|Texas Instruments Incorporated
| IBIS Model of : TMUX7211
| 48V 4x1:1 Analog Switch Array
| This file contains package information for the following:
|  TSSOP 16-pin (PW) package as [Component] TMUX7211_PW
|  QFN 16-pin (RUM) package as [Component] TMUX7211_RUM
| This device can be powered at the following Vccs:
| Single Rail Supply Configurations:
|  5.0 volt VDD, 0V VSS
|  12.0 volt VDD, 0V VSS
|  36.0 volt VDD, 0V VSS
|  44.0 volt VDD, 0V VSS
| Dual Rail Supply Configurations:
|  5.0 volt VDD, -5V VSS
|  15.0 volt VDD, -15V VSS
|  20.0 volt VDD, -20V VSS
| Digital Voltage Range : 4.5-48.4
[IBIS Ver] 4.1
[File name] tmux7211.ibs
[File Rev] 1.0
[Date] 12/09/2020
[Source]
| Texas Instruments Incorporated.
| 12500 TI Blvd
| Dallas, TX -75243
[Notes] Revision History:
| Rev 1.0: 12/09/2020
| - Initial version of the model
| - Model generated from simulations in TISPICE/SPECTRE
| - C_comp although listed in numerical order of value are
| obtained from varying PVT conditions. For PVT conditions for
| each specific value refer the buffer description under
| respective [Model]. IBIS model user is responsible for using
| appropriate C_comp to simulate for Signal Integrity.
| - Warnings regarding combined Non-monotonicity of various models have been
| reviewed and considered minor and can be ignored.
|**** Modify the following if you use [Model Selector]***********
| - Model names with a trailing voltage extension contain the model for
| operation at that voltage range.
[Disclaimer]
| This model is designed as an aid for customers of Texas Instruments.
| TI and its licensors and suppliers make no warranties, either expressed
| or implied, with respect to this model, including the warranties of
| merchantability or fitness for a particular purpose. The model is
| provided solely on an "as is" basis. The entire risk as to its quality
| and performance is with the customer.
| This model is subject to change without notice. Texas Instruments
| Incorporated is not responsible for updating this model.
[Copyright]
(C) Copyright 2020 Texas Instruments Incorporated. All rights reserved.
| Component TMUX7211_DGK 8-pin SOT (per package)
[Component] TMUX7211_PW
[Manufacturer]  Texas Instruments Incorporated
[Package] |TSSOP (PW) 16-pin
| variable typ min max
R_pkg 0.05 0.04 0.06
L_pkg 1.0nH 0.8nH 1.2nH
C_pkg 0.2pF 0.16pF 0.24pF
| pin number (pin name) mapping to model name
[Pin] signal_name   model_name   R_pin L_pin C_pin
1   IN1 		INPUT_PD   NA   NA   NA
2   D1   TMUX7211_DX   NA   NA   NA
3   S1   TMUX7211_SX   NA   NA   NA
4   VSS   POWER   NA   NA   NA
5   GND 		GND   NA   NA   NA
6   S4   TMUX7211_SX   NA   NA   NA
7   D4   TMUX7211_DX   NA   NA   NA
8   IN4 		INPUT_PD   NA   NA   NA
9   IN3 		INPUT_PD   NA   NA   NA
10   D3   TMUX7211_DX   NA   NA   NA
11   S3   TMUX7211_SX   NA   NA   NA
12   NC   NC   NA   NA   NA
13   VDD 		POWER   NA   NA   NA
14   S2   TMUX7211_SX   NA   NA   NA
15   D2   TMUX7211_DX   NA   NA   NA
16   IN2 		INPUT_PD   NA   NA   NA
[Series Switch Groups]
| Function Group States
On  1 /   | S1->D1 IN HIGH
Off  /   | EN LOW
[Series Pin Mapping]   pin_2   model_name   function_table_group
| PW Package
|2   3   TMUX7211_SX_SINGLE_5V_S   1
|3   2   TMUX7211_DX_SINGLE_5V_S   1
|15   14   TMUX7211_SX_SINGLE_5V_S   1
|14   15   TMUX7211_DX_SINGLE_5V_S   1
|7   6   TMUX7211_SX_SINGLE_5V_S   1
|6   7   TMUX7211_DX_SINGLE_5V_S   1
|10   11   TMUX7211_SX_SINGLE_5V_S   1
|11   10   TMUX7211_DX_SINGLE_5V_S   1
|2   3   TMUX7211_SX_SINGLE_12V_S   1
|3   2   TMUX7211_DX_SINGLE_12V_S   1
|15   14   TMUX7211_SX_SINGLE_12V_S   1
|14   15   TMUX7211_DX_SINGLE_12V_S   1
|7   6   TMUX7211_SX_SINGLE_12V_S   1
|6   7   TMUX7211_DX_SINGLE_12V_S   1
|10   11   TMUX7211_SX_SINGLE_12V_S   1
|11   10   TMUX7211_DX_SINGLE_12V_S   1
|2   3   TMUX7211_SX_SINGLE_36V_S   1
|3   2   TMUX7211_DX_SINGLE_36V_S   1
|15   14   TMUX7211_SX_SINGLE_36V_S   1
|14   15   TMUX7211_DX_SINGLE_36V_S   1
|7   6   TMUX7211_SX_SINGLE_36V_S   1
|6   7   TMUX7211_DX_SINGLE_36V_S   1
|10   11   TMUX7211_SX_SINGLE_36V_S   1
|11   10   TMUX7211_DX_SINGLE_36V_S   1
2   3   TMUX7211_SX_SINGLE_44V_S   1
3   2   TMUX7211_DX_SINGLE_44V_S   1
15   14   TMUX7211_SX_SINGLE_44V_S   1
14   15   TMUX7211_DX_SINGLE_44V_S   1
7   6   TMUX7211_SX_SINGLE_44V_S   1
6   7   TMUX7211_DX_SINGLE_44V_S   1
10   11   TMUX7211_SX_SINGLE_44V_S   1
11   10   TMUX7211_DX_SINGLE_44V_S   1
|2   3   TMUX7211_SX_DUAL_PM5_S   1
|3   2   TMUX7211_DX_DUAL_PM5_S   1
|15   14   TMUX7211_SX_DUAL_PM5_S   1
|14   15   TMUX7211_DX_DUAL_PM5_S   1
|7   6   TMUX7211_SX_DUAL_PM5_S   1
|6   7   TMUX7211_DX_DUAL_PM5_S   1
|10   11   TMUX7211_SX_DUAL_PM5_S   1
|11   10   TMUX7211_DX_DUAL_PM5_S   1
|2   3   TMUX7211_SX_DUAL_PM15_S   1
|3   2   TMUX7211_DX_DUAL_PM15_S   1
|15   14   TMUX7211_SX_DUAL_PM15_S   1
|14   15   TMUX7211_DX_DUAL_PM15_S   1
|7   6   TMUX7211_SX_DUAL_PM15_S   1
|6   7   TMUX7211_DX_DUAL_PM15_S   1
|10   11   TMUX7211_SX_DUAL_PM15_S   1
|11   10   TMUX7211_DX_DUAL_PM15_S   1
|2   3   TMUX7211_SX_DUAL_PM20_S   1
|3   2   TMUX7211_DX_DUAL_PM20_S   1
|15   14   TMUX7211_SX_DUAL_PM20_S   1
|14   15   TMUX7211_DX_DUAL_PM20_S   1
|7   6   TMUX7211_SX_DUAL_PM20_S   1
|6   7   TMUX7211_DX_DUAL_PM20_S   1
|10   11   TMUX7211_SX_DUAL_PM20_S   1
|11   10   TMUX7211_DX_DUAL_PM20_S   1
| Component TMUX7211_RUM 16-pin QFN (per package)
[Component] TMUX7211_RUM
[Manufacturer]  Texas Instruments Incorporated
[Package] |QFN (RUM) 16-pin
| variable typ 		min 		max
R_pkg 	0.05 		0.04 		0.06
L_pkg 	1.0nH 	0.8nH 	1.2nH
C_pkg 	0.2pF 	0.16pF 	0.24pF
| pin number (pin name) mapping to model name
[Pin] signal_name   model_name   R_pin L_pin C_pin
1   S1   TMUX7211_SX   NA   NA   NA
2   VSS   POWER   NA   NA   NA
3   GND 		GND   NA   NA   NA
4   S4   TMUX7211_SX   NA   NA   NA
5   D4   TMUX7211_DX   NA   NA   NA
6   IN4 		INPUT_PD   NA   NA   NA
7   IN3 		INPUT_PD   NA   NA   NA
8   D3   TMUX7211_DX   NA   NA   NA
9   S3   TMUX7211_SX   NA   NA   NA
10   NC   NC   NA   NA   NA
11   VDD 		POWER   NA   NA   NA
12   S2   TMUX7211_SX   NA   NA   NA
13   D2   TMUX7211_DX   NA   NA   NA
14   IN2 		INPUT_PD   NA   NA   NA
15   IN1 		INPUT_PD   NA   NA   NA
16   D1   TMUX7211_DX   NA   NA   NA
[Series Switch Groups]
| Function Group States
|On  1 /   | S1->D1 IN HIGH
|Off  /   | EN LOW
[Series Pin Mapping]   pin_2   model_name   function_table_group
| RUM Package
|16   1   TMUX7211_SX_SINGLE_5V_S   1
|1   16   TMUX7211_DX_SINGLE_5V_S   1
|13   12   TMUX7211_SX_SINGLE_5V_S   1
|12   13   TMUX7211_DX_SINGLE_5V_S   1
|8   8   TMUX7211_SX_SINGLE_5V_S   1
|9   9   TMUX7211_DX_SINGLE_5V_S   1
|5   4   TMUX7211_SX_SINGLE_5V_S   1
|4   5   TMUX7211_DX_SINGLE_5V_S   1
|16   1   TMUX7211_SX_SINGLE_12V_S   1
|1   16   TMUX7211_DX_SINGLE_12V_S   1
|13   12   TMUX7211_SX_SINGLE_12V_S   1
|12   13   TMUX7211_DX_SINGLE_12V_S   1
|8   8   TMUX7211_SX_SINGLE_12V_S   1
|9   9   TMUX7211_DX_SINGLE_12V_S   1
|5   4   TMUX7211_SX_SINGLE_12V_S   1
|4   5   TMUX7211_DX_SINGLE_12V_S   1
|16   1   TMUX7211_SX_SINGLE_36V_S   1
|1   16   TMUX7211_DX_SINGLE_36V_S   1
|13   12   TMUX7211_SX_SINGLE_36V_S   1
|12   13   TMUX7211_DX_SINGLE_36V_S   1
|8   8   TMUX7211_SX_SINGLE_36V_S   1
|9   9   TMUX7211_DX_SINGLE_36V_S   1
|5   4   TMUX7211_SX_SINGLE_36V_S   1
|4   5   TMUX7211_DX_SINGLE_36V_S   1
|16   1   TMUX7211_SX_SINGLE_44V_S   1
|1   16   TMUX7211_DX_SINGLE_44V_S   1
|13   12   TMUX7211_SX_SINGLE_44V_S   1
|12   13   TMUX7211_DX_SINGLE_44V_S   1
|8   8   TMUX7211_SX_SINGLE_44V_S   1
|9   9   TMUX7211_DX_SINGLE_44V_S   1
|5   4   TMUX7211_SX_SINGLE_44V_S   1
|4   5   TMUX7211_DX_SINGLE_44V_S   1
|16   1   TMUX7211_SX_DUAL_PM5_S   1
|1   16   TMUX7211_DX_DUAL_PM5_S   1
|13   12   TMUX7211_SX_DUAL_PM5_S   1
|12   13   TMUX7211_DX_DUAL_PM5_S   1
|8   8   TMUX7211_SX_DUAL_PM5_S   1
|9   9   TMUX7211_DX_DUAL_PM5_S   1
|5   4   TMUX7211_SX_DUAL_PM5_S   1
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[Model Selector] INPUT_PU
INBUF_PU_5V   INPUT_PU   buffer at 5V operation.
INBUF_PU_12V   INPUT_PU   buffer at 12V operation.
INBUF_PU_15V   INPUT_PU   buffer at 15V operation.
INBUF_PU_20V   INPUT_PU   buffer at 20V operation.
INBUF_PU_36V   INPUT_PU   buffer at 36V operation.
INBUF_PU_44V   INPUT_PU   buffer at 44V operation.
[Model Selector] INPUT_PD
INBUF_PD_5V   INPUT_PD   buffer at 5V operation.
INBUF_PD_12V   INPUT_PD   buffer at 12V operation.
INBUF_PD_15V   INPUT_PD   buffer at 15V operation.
INBUF_PD_20V   INPUT_PD   buffer at 20V operation.
INBUF_PD_36V   INPUT_PD   buffer at 36V operation.
INBUF_PD_44V   INPUT_PD   buffer at 44V operation.
[Model Selector] TMUX7211_SX
TMUX7211_SX_SINGLE_5V  switch termination at +5V operation.
TMUX7211_SX_SINGLE_12V  switch termination at +12V operation.
TMUX7211_SX_SINGLE_36V  switch termination at +36V operation.
TMUX7211_SX_SINGLE_44V  switch termination at +44V operation.
TMUX7211_SX_DUAL_PM5  switch termination at +/-5V operation.
TMUX7211_SX_DUAL_PM15  switch termination at +/-15V operation.
TMUX7211_SX_DUAL_PM20  switch termination at +/-20V operation.
[Model Selector] TMUX7211_SX_S
TMUX7211_SX_SINGLE_5V_S  switch at +5V operation.
TMUX7211_SX_SINGLE_12V_S  switch at +12V operation.
TMUX7211_SX_SINGLE_36V_S  switch at +36V operation.
TMUX7211_SX_SINGLE_44V_S  switch at +44V operation.
TMUX7211_SX_DUAL_PM5_S  switch at +/-5V operation.
TMUX7211_SX_DUAL_PM15_S  switch at +/-15V operation.
TMUX7211_SX_DUAL_PM20_S  switch at +/-20V operation.
[Model Selector] TMUX7211_DX
TMUX7211_DX_SINGLE_5V  termination switch at +5V operation.
TMUX7211_DX_SINGLE_12V  termination switch at +12V operation.
TMUX7211_DX_SINGLE_36V  termination switch at +36V operation.
TMUX7211_DX_SINGLE_44V  termination switch at +44V operation.
TMUX7211_DX_DUAL_PM5  termination switch at +/-5V operation.
TMUX7211_DX_DUAL_PM15  termination switch at +/-15V operation.
TMUX7211_DX_DUAL_PM20  termination switch at +/-20V operation.
[Model Selector] TMUX7211_DX_S
TMUX7211_DX_SINGLE_5V_S  switch at +5V operation.
TMUX7211_DX_SINGLE_12V_S  switch at +12V operation.
TMUX7211_DX_SINGLE_36V_S  switch at +36V operation.
TMUX7211_DX_SINGLE_44V_S  switch at +44V operation.
TMUX7211_DX_DUAL_PM5_S  switch at +/-5V operation.
TMUX7211_DX_DUAL_PM15_S  switch at +/-15V operation.
TMUX7211_DX_DUAL_PM20_S  switch at +/-20V operation.
[Model]   TMUX7211_SX_SINGLE_5V_S
Model_type  Series_switch
| variable   typ   min   max
C_comp   0   0   0
[Temperature Range]   25   125   -40
| Ambient temperature   25   125   -40
[Voltage range]   5   4.5   5.5
[On]
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[Off]
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[Model]   TMUX7211_DX_SINGLE_5V_S
Model_type  Series_switch
| variable   typ   min   max
C_comp   0   0   0
[Temperature Range]   25   125   -40
| Ambient temperature   25   125   -40
[Voltage range]   5   5   5
[On]
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[Off]
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[Model]   TMUX7211_SX_SINGLE_12V_S
Model_type  Series_switch
| variable   typ   min   max
C_comp   0   0   0
[Temperature Range]   25   125   -40
| Ambient temperature   25   125   -40
[Voltage range]   12   12   12
[On]
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[Off]
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[Model]   TMUX7211_DX_SINGLE_12V_S
Model_type  Series_switch
| variable   typ   min   max
C_comp   0   0   0
[Temperature Range]   25   125   -40
| Ambient temperature   25   125   -40
[Voltage range]   12   12   12
[On]
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[Off]
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[Model]   TMUX7211_SX_SINGLE_36V_S
Model_type  Series_switch
| variable   typ   min   max
C_comp   0   0   0
[Temperature Range]   25   125   -40
| Ambient temperature   25   125   -40
[Voltage range]   36   36   36
[On]
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[Off]
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[Model]   TMUX7211_DX_SINGLE_36V_S
Model_type  Series_switch
| variable   typ   min   max
C_comp   0   0   0
[Temperature Range]   25   125   -40
| Ambient temperature   25   125   -40
[Voltage range]   36   36   36
[On]
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[Off]
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[Model]   TMUX7211_SX_SINGLE_44V_S
Model_type  Series_switch
| variable   typ   min   max
C_comp   0   0   0
[Temperature Range]   25   125   -40
| Ambient temperature   25   125   -40
[Voltage range]   44   44   44
[On]
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[Off]
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[Model]   TMUX7211_DX_SINGLE_44V_S
Model_type  Series_switch
| variable   typ   min   max
C_comp   0   0   0
[Temperature Range]   25   125   -40
| Ambient temperature   25   125   -40
[Voltage range]   44   44   44
[On]
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[Off]
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[Model]   TMUX7211_SX_DUAL_PM5_S
Model_type  Series_switch
| variable   typ   min   max
C_comp   0   0   0
[Temperature Range]   25   125   -40
| Ambient temperature   25   125   -40
[Voltage range]   0   -5   5
[On]
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[Off]
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[Model]   TMUX7211_DX_DUAL_PM5_S
Model_type  Series_switch
| variable   typ   min   max
C_comp   0   0   0
[Temperature Range]   25   125   -40
| Ambient temperature   25   125   -40
[Voltage range]   0   -5   5
[On]
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[Off]
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[Model]   TMUX7211_SX_DUAL_PM15_S
Model_type  Series_switch
| variable   typ   min   max
C_comp   0   0   0
[Temperature Range]   25   125   -40
| Ambient temperature   25   125   -40
[Voltage range]   0   -15   15
[On]
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[Off]
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[Model]   TMUX7211_DX_DUAL_PM15_S
Model_type  Series_switch
| variable   typ   min   max
C_comp   0   0   0
[Temperature Range]   25   125   -40
| Ambient temperature   25   125   -40
[Voltage range]   0   -15   15
[On]
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[Off]
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[Model]   TMUX7211_SX_DUAL_PM20_S
Model_type  Series_switch
| variable   typ   min   max
C_comp   0   0   0
[Temperature Range]   25   125   -40
| Ambient temperature   25   125   -40
[Voltage range]   0   -20   20
[On]
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[Off]
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[Model]   TMUX7211_DX_DUAL_PM20_S
Model_type  Series_switch
| variable   typ   min   max
C_comp   0   0   0
[Temperature Range]   25   125   -40
| Ambient temperature   25   125   -40
[Voltage range]   0   -20   20
[On]
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[Off]
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| Models and submodels in the file (40): INBUF_PD_5V (Input), INBUF_PD_12V (Input), INBUF_PD_15V (Input), INBUF_PD_20V (Input), INBUF_PD_36V (Input), INBUF_PD_44V (Input), INBUF_PU_5V (Input), INBUF_PU_12V (Input), INBUF_PU_15V (Input), INBUF_PU_20V (Input), INBUF_PU_36V (Input), INBUF_PU_44V (Input), TMUX7211_SX_SINGLE_5V_S (Series_switch), TMUX7211_SX_SINGLE_5V (Terminator), TMUX7211_DX_SINGLE_5V_S (Series_switch), TMUX7211_DX_SINGLE_5V (Terminator), TMUX7211_SX_SINGLE_12V_S (Series_switch), TMUX7211_SX_SINGLE_12V (Terminator), TMUX7211_DX_SINGLE_12V_S (Series_switch), TMUX7211_DX_SINGLE_12V (Terminator), TMUX7211_SX_SINGLE_36V_S (Series_switch), TMUX7211_SX_SINGLE_36V (Terminator), TMUX7211_DX_SINGLE_36V_S (Series_switch), TMUX7211_DX_SINGLE_36V (Terminator), TMUX7211_SX_SINGLE_44V_S (Series_switch), TMUX7211_SX_SINGLE_44V (Terminator), TMUX7211_DX_SINGLE_44V_S (Series_switch), TMUX7211_DX_SINGLE_44V (Terminator), TMUX7211_SX_DUAL_PM5_S (Series_switch), TMUX7211_SX_DUAL_PM5 (Terminator), TMUX7211_DX_DUAL_PM5_S (Series_switch), TMUX7211_DX_DUAL_PM5 (Terminator), TMUX7211_SX_DUAL_PM15_S (Series_switch), TMUX7211_SX_DUAL_PM15 (Terminator), TMUX7211_DX_DUAL_PM15_S (Series_switch), TMUX7211_DX_DUAL_PM15 (Terminator), TMUX7211_SX_DUAL_PM20_S (Series_switch), TMUX7211_SX_DUAL_PM20 (Terminator), TMUX7211_DX_DUAL_PM20_S (Series_switch), TMUX7211_DX_DUAL_PM20 (Terminator)
